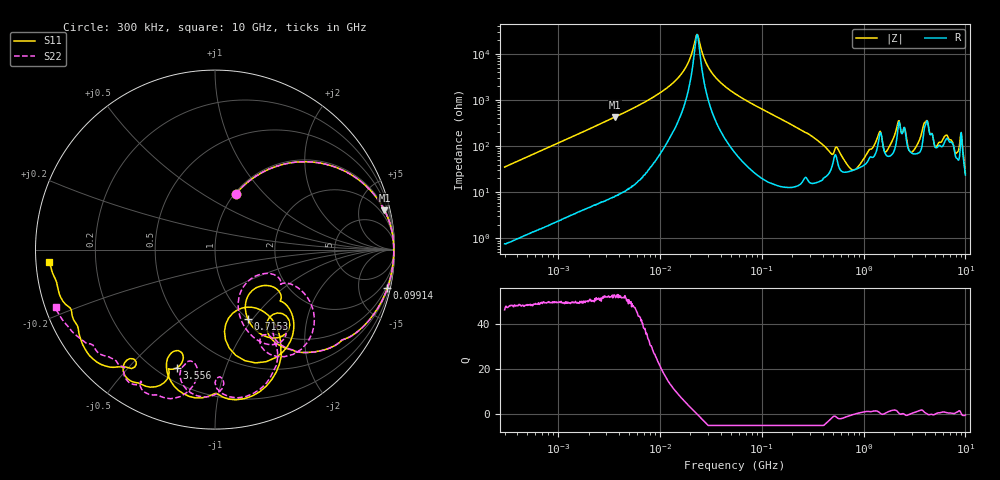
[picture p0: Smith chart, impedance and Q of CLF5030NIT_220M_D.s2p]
! S-Parameter Data Generated by TDK Corporation
! Copyright(C) 2019 TDK Corporation.
! All Rights Reserved.
! TDK P/N: CLF5030NIT-220M-D (Inductor)
! Property: L=22uH at 100kHz
! Size(LxWxT): 5.3x5x2.7mm
! Model Type: s2p (Touchstone File Format Version 1.0)
! Frequency: DC=Yes Start=0.3MHz Stop=10000MHz 802points Log-sweep
! Model Generated on May 10, 2019
! Port Assignments:
!  1 ---@@@--- 2
! Applicable Conditions:
!  Temperature = 25 degC
!  DC Bias Current = 0 A
!  Small Signal Operation
! Terms and conditions regarding TDK Simulation Models
! (1)This simulation model is being provided solely for informational purposes. Please refer to the specifications of the products in terms of detailed characteristics of such products.
! (2)In no event shall TDK Corporation of any of its subsidiaries be liable for any loss or damage arising, directly or indirectly,
!  From any information contained in this simulation model, including, but not limited to loss or damages arising from any inaccuracies, omissions or errors in connection with such information.
! (3)Any and all copyrights on this simulation model are owned by TDK Corporation.
!  Duplication or redistribution of this simulation model without prior written permission from TDK Corporation is prohibited.
! (4)This simulation model is subject to any modification or change without any prior notice.
! (5)Neither TDK Corporation nor any of its subsidiaries shall make any warranty, express or implied,
!  Including but not limited to the correctness, implied warranties of merchantability and fitness for a particular purpose with respect to this simulation models.
! (6)The use of this simulation model shall be deemed to have consented to the terms and conditions hereof.
# Hz S MA R 50
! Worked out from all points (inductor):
!   801 points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, 300 kHz to 10 GHz, reference 50 ohm
!   read as one part in series: L = 18.7 uH near 318.3 kHz
!   highest Q = 52.5 at 3.599 MHz (marker M1), where L = 18.7 uH
!   self-resonance near 23.15 MHz
!   S11 on the Smith chart (normalised r, x): 300 kHz: 1.01, +0.71; 99.14 MHz: 0.67, -8.96; 715.3 MHz: 1.00, -0.95; 3.556 GHz: 0.27, -0.69; 10 GHz: 0.04, -0.04
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300000  0.3318 69.4  0.9363 -19.3  0.9361 -19.3  0.3318 69.5
1713600  0.8863 26.4  0.4454 -62.5  0.4453 -62.4  0.8865 26.4
3598556  0.969 13.1  0.2293 -75.8  0.2293 -75.8  0.969 13.1
9671944  0.9941 3.8  0.07345 -83.7  0.07346 -83.7  0.9941 3.8
1.694973e7  0.9959 0.7  0.02402 -80.4  0.02404 -80.4  0.996 0.7
2.315417e7  0.9962 -0.9  0.003768 -6.0  0.003768 -6.0  0.9963 -0.9
3.206042e7  0.9959 -2.7  0.02446 78.6  0.02449 78.6  0.996 -2.7
5.477226e7  0.9935 -6.3  0.07193 80.6  0.07195 80.6  0.9937 -6.4
9.914192e7  0.9838 -12.7  0.1505 75.5  0.1505 75.5  0.984 -12.8
3.126428e8  0.8383 -41.1  0.475 43.8  0.475 43.8  0.8387 -41.1
7.152593e8  0.4272 -64.7  0.7156 -7.7  0.7158 -7.7  0.4035 -69.6
1.069912e9  0.3758 -33.0  0.6566 -50.1  0.657 -50.2  0.3204 -24.4
1.459486e9  0.6867 -65.4  0.2703 -64.5  0.2705 -64.7  0.7297 -44.9
1.767019e9  0.3997 -54.8  0.5122 -77.7  0.5122 -77.8  0.5589 -58.4
2.264206e9  0.8448 -82.1  0.1449 -79.5  0.1444 -80.2  0.8021 -87.3
3.008786e9  0.6109 -112.0  0.3453 -88.4  0.3429 -88.5  0.6445 -104.0
3.556288e9  0.6926 -108.0  0.2208 -139.2  0.2172 -139.0  0.7625 -99.0
4.107799e9  0.7701 -110.3  0.07921 -118.3  0.0803 -117.1  0.8732 -112.1
5.21579e9  0.7588 -126.1  0.1784 -119.0  0.179 -118.9  0.8268 -127.5
8.09931e9  0.8698 -158.0  0.06254 -163.6  0.06321 -163.9  0.9281 -153.3
9.217363e9  0.9031 -169.1  0.01203 -112.9  0.01185 -116.4  0.9454 -159.0
1e10  0.9257 -175.8  0.03336 -88.1  0.03289 -87.4  0.941 -160.1
